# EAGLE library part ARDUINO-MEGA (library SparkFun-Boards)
Arduino Mega board footprint
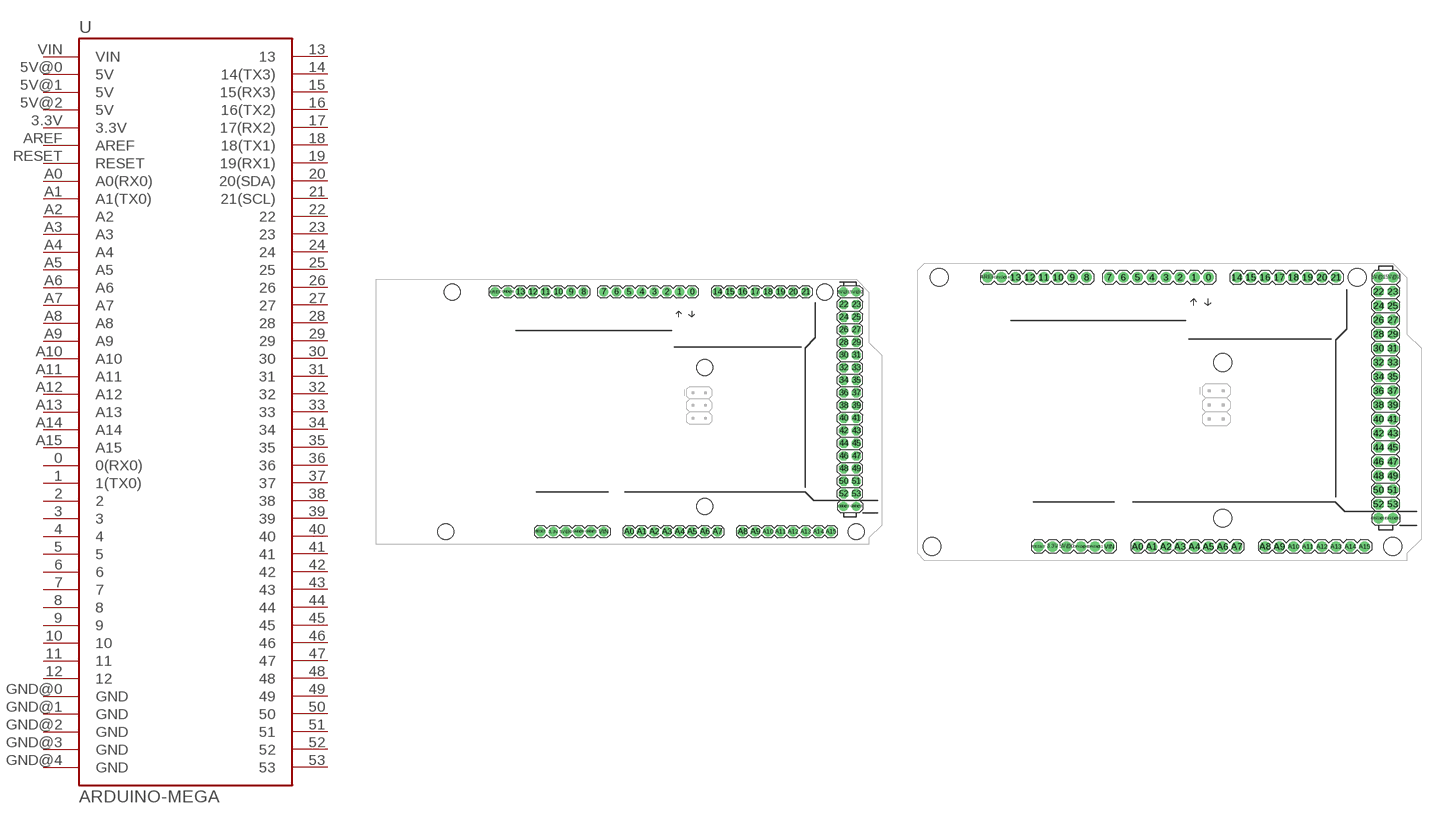
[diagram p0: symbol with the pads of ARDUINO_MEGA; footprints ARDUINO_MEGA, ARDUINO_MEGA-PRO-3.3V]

Designator prefix U

## ARDUINO-MEGAFULL  [ARDUINO_MEGA]
0  0(RX0)
1  1(TX0)
2  2
3  3
3.3V  3.3V
4  4
5  5
5V@0  5V
5V@1  5V
5V@2  5V
6  6
7  7
8  8
9  9
10  10
11  11
12  12
13  13
14  14(TX3)
15  15(RX3)
16  16(TX2)
17  17(RX2)
18  18(TX1)
19  19(RX1)
20  20(SDA)
21  21(SCL)
22  22
23  23
24  24
25  25
26  26
27  27
28  28
29  29
30  30
31  31
32  32
33  33
34  34
35  35
36  36
37  37
38  38
39  39
40  40
41  41
42  42
43  43
44  44
45  45
46  46
47  47
48  48
49  49
50  50
51  51
52  52
53  53
A0  A0(RX0)
A1  A1(TX0)
A2  A2
A3  A3
A4  A4
A5  A5
A6  A6
A7  A7
A8  A8
A9  A9
A10  A10
A11  A11
A12  A12
A13  A13
A14  A14
A15  A15
AREF  AREF
GND@0  GND
GND@1  GND
GND@2  GND
GND@3  GND
GND@4  GND
RESET  RESET
VIN  VIN

## ARDUINO-MEGAPRO  [ARDUINO_MEGA-PRO-3.3V]
Pads as for ARDUINO_MEGA

## ARDUINO-MEGAPRO-5V  [ARDUINO_MEGA-PRO-5V]
Pads as for ARDUINO_MEGA

## Footprint ARDUINO_MEGA (pad centres in mm)
Full Arduino MEGA footprint
drill 1.016 pad 1.88: 0 63.5,50.8; 1 60.96,50.8; 2 58.42,50.8; 3 55.88,50.8; 3.3V 35.56,2.54; 4 53.34,50.8; 5 50.8,50.8; 5V@0 38.1,2.54; 5V@1 93.98,50.8; 5V@2 96.52,50.8; 6 48.26,50.8; 7 45.72,50.8; 8 41.656,50.8; 9 39.116,50.8; 10 36.576,50.8; 11 34.036,50.8; 12 31.496,50.8; 13 28.956,50.8; 14 68.58,50.8; 15 71.12,50.8; 16 73.66,50.8; 17 76.2,50.8; 18 78.74,50.8; 19 81.28,50.8; 20 83.82,50.8; 21 86.36,50.8; A0 50.8,2.54; A1 53.34,2.54; A2 55.88,2.54; A3 58.42,2.54; A4 60.96,2.54; A5 63.5,2.54; A6 66.04,2.54; A7 68.58,2.54; A8 73.66,2.54; A9 76.2,2.54; A10 78.74,2.54; A11 81.28,2.54; A12 83.82,2.54; A13 86.36,2.54; A14 88.9,2.54; A15 91.44,2.54; AREF 23.876,50.8; GND@0 40.64,2.54; GND@1 43.18,2.54; GND@2 93.98,7.62; GND@3 96.52,7.62; GND@4 26.416,50.8; RESET 33.02,2.54; VIN 45.72,2.54
drill 1.016 pad 1.88 octagon: 22 93.98,48.26; 23 96.52,48.26; 24 93.98,45.72; 25 96.52,45.72; 26 93.98,43.18; 27 96.52,43.18; 28 93.98,40.64; 29 96.52,40.64; 30 93.98,38.1; 31 96.52,38.1; 32 93.98,35.56; 33 96.52,35.56; 34 93.98,33.02; 35 96.52,33.02; 36 93.98,30.48; 37 96.52,30.48; 38 93.98,27.94; 39 96.52,27.94; 40 93.98,25.4; 41 96.52,25.4; 42 93.98,22.86; 43 96.52,22.86; 44 93.98,20.32; 45 96.52,20.32; 46 93.98,17.78; 47 96.52,17.78; 48 93.98,15.24; 49 96.52,15.24; 50 93.98,12.7; 51 96.52,12.7; 52 93.98,10.16; 53 96.52,10.16
hole 3.2 at 15.24,50.8
hole 3.2 at 13.97,2.54
hole 3.2 at 66.04,35.56
hole 3.2 at 66.04,7.62
hole 3.2 at 90.17,50.8
hole 3.2 at 96.52,2.54

## Footprint ARDUINO_MEGA-PRO-3.3V (pad centres in mm)
Arduino Mega Pro footprint
drill 1.016 pad 1.88: 0 52.07,50.8; 1 49.53,50.8; 2 46.99,50.8; 3 44.45,50.8; 3.3V 24.13,2.54; 4 41.91,50.8; 5 39.37,50.8; 5V@0 26.67,2.54; 5V@1 82.55,50.8; 5V@2 85.09,50.8; 6 36.83,50.8; 7 34.29,50.8; 8 30.226,50.8; 9 27.686,50.8; 10 25.146,50.8; 11 22.606,50.8; 12 20.066,50.8; 13 17.526,50.8; 14 57.15,50.8; 15 59.69,50.8; 16 62.23,50.8; 17 64.77,50.8; 18 67.31,50.8; 19 69.85,50.8; 20 72.39,50.8; 21 74.93,50.8; A0 39.37,2.54; A1 41.91,2.54; A2 44.45,2.54; A3 46.99,2.54; A4 49.53,2.54; A5 52.07,2.54; A6 54.61,2.54; A7 57.15,2.54; A8 62.23,2.54; A9 64.77,2.54; A10 67.31,2.54; A11 69.85,2.54; A12 72.39,2.54; A13 74.93,2.54; A14 77.47,2.54; A15 80.01,2.54; AREF 12.446,50.8; GND@0 29.21,2.54; GND@1 31.75,2.54; GND@2 82.55,7.62; GND@3 85.09,7.62; GND@4 14.986,50.8; RESET 21.59,2.54; VIN 34.29,2.54
drill 1.016 pad 1.88 octagon: 22 82.55,48.26; 23 85.09,48.26; 24 82.55,45.72; 25 85.09,45.72; 26 82.55,43.18; 27 85.09,43.18; 28 82.55,40.64; 29 85.09,40.64; 30 82.55,38.1; 31 85.09,38.1; 32 82.55,35.56; 33 85.09,35.56; 34 82.55,33.02; 35 85.09,33.02; 36 82.55,30.48; 37 85.09,30.48; 38 82.55,27.94; 39 85.09,27.94; 40 82.55,25.4; 41 85.09,25.4; 42 82.55,22.86; 43 85.09,22.86; 44 82.55,20.32; 45 85.09,20.32; 46 82.55,17.78; 47 85.09,17.78; 48 82.55,15.24; 49 85.09,15.24; 50 82.55,12.7; 51 85.09,12.7; 52 82.55,10.16; 53 85.09,10.16
hole 3.2 at 3.81,50.8
hole 3.2 at 2.54,2.54
hole 3.2 at 54.61,35.56
hole 3.2 at 54.61,7.62
hole 3.2 at 78.74,50.8
hole 3.2 at 85.09,2.54

## Footprint ARDUINO_MEGA-PRO-5V (pad centres in mm)
drill 1.016 pad 1.88: 0 52.07,50.8; 1 49.53,50.8; 2 46.99,50.8; 3 44.45,50.8; 3.3V 24.13,2.54; 4 41.91,50.8; 5 39.37,50.8; 5V@0 26.67,2.54; 5V@1 82.55,50.8; 5V@2 85.09,50.8; 6 36.83,50.8; 7 34.29,50.8; 8 30.226,50.8; 9 27.686,50.8; 10 25.146,50.8; 11 22.606,50.8; 12 20.066,50.8; 13 17.526,50.8; 14 57.15,50.8; 15 59.69,50.8; 16 62.23,50.8; 17 64.77,50.8; 18 67.31,50.8; 19 69.85,50.8; 20 72.39,50.8; 21 74.93,50.8; A0 39.37,2.54; A1 41.91,2.54; A2 44.45,2.54; A3 46.99,2.54; A4 49.53,2.54; A5 52.07,2.54; A6 54.61,2.54; A7 57.15,2.54; A8 62.23,2.54; A9 64.77,2.54; A10 67.31,2.54; A11 69.85,2.54; A12 72.39,2.54; A13 74.93,2.54; A14 77.47,2.54; A15 80.01,2.54; AREF 12.446,50.8; GND@0 29.21,2.54; GND@1 31.75,2.54; GND@2 82.55,7.62; GND@3 85.09,7.62; GND@4 14.986,50.8; RESET 21.59,2.54; VIN 34.29,2.54
drill 1.016 pad 1.88 octagon: 22 82.55,48.26; 23 85.09,48.26; 24 82.55,45.72; 25 85.09,45.72; 26 82.55,43.18; 27 85.09,43.18; 28 82.55,40.64; 29 85.09,40.64; 30 82.55,38.1; 31 85.09,38.1; 32 82.55,35.56; 33 85.09,35.56; 34 82.55,33.02; 35 85.09,33.02; 36 82.55,30.48; 37 85.09,30.48; 38 82.55,27.94; 39 85.09,27.94; 40 82.55,25.4; 41 85.09,25.4; 42 82.55,22.86; 43 85.09,22.86; 44 82.55,20.32; 45 85.09,20.32; 46 82.55,17.78; 47 85.09,17.78; 48 82.55,15.24; 49 85.09,15.24; 50 82.55,12.7; 51 85.09,12.7; 52 82.55,10.16; 53 85.09,10.16
hole 3.2 at 3.81,50.8
hole 3.2 at 2.54,2.54
hole 3.2 at 54.61,35.56
hole 3.2 at 54.61,7.62
hole 3.2 at 78.74,50.8
hole 3.2 at 85.09,2.54

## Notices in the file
Licensing: Creative Commons ShareAlike 4.0 International - https://creativecommons.org/licenses/by-sa/4.0
